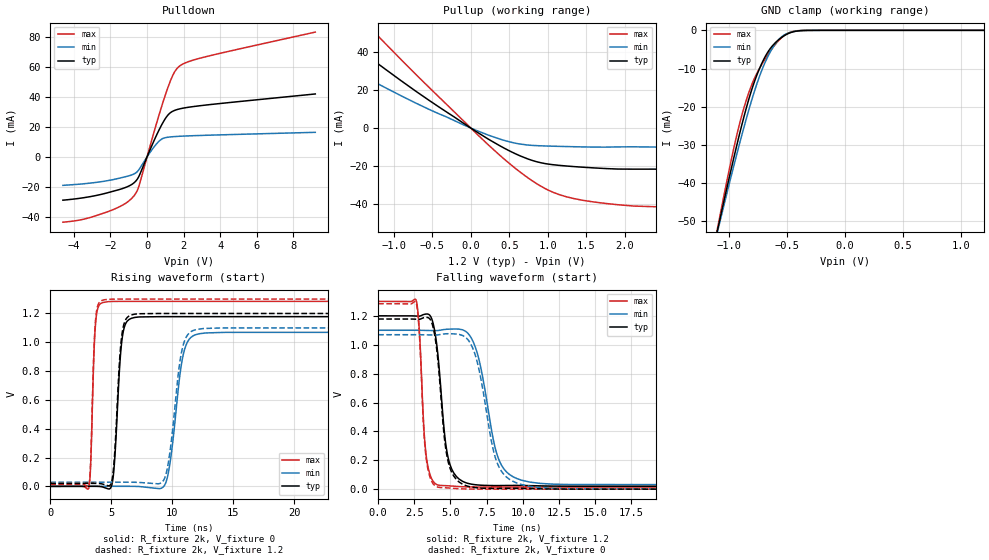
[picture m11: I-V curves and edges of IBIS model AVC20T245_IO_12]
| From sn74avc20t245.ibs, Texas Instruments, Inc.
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[Model]   AVC20T245_IO_12
Model_type  I/O
Vinl=0.385
Vinh=0.845
Enable   Active-Low
Vref =   0
Rref =   2000
Cref =   15p
Vmeas =   0.6
| variable   typ   min   max
C_comp   5.29pF   4.66pF   5.83pF
| C_pullup   5.78pF   3.89pF   7.84pF
| C_pulldown   5.32pF   4.76pF   7.02pF
| C_tri-state   5.29pF   4.66pF   5.83pF
[Temperature Range]   40   100   -40
| Ambient temperature   25   85   -40
[Voltage range]   1.2   1.1   1.3
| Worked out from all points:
|   slope of the pulldown table from 0 to 0.18 V, typ, clamps not added: 34.6 ohm
|   slope of the pullup table from 0 to 0.18 V, typ, clamps not added: 38.6 ohm
|   GND clamp passes 1 mA (typ) near -0.50 V on its own axis
|   rising waveform, R_fixture 2k, V_fixture 0: 20-80 % time 468ps typ, 865ps min, 281ps max; typ from 0 V to 1.18 V
|   falling waveform, R_fixture 2k, V_fixture 1.2: 20-80 % time 670ps typ, 1.21ns min, 399ps max; typ from 1.2 V to 0.02 V
|   rising waveform, R_fixture 2k, V_fixture 1.2: 20-80 % time 463ps typ, 848ps min, 279ps max; typ from 0.02 V to 1.2 V
|   falling waveform, R_fixture 2k, V_fixture 0: 20-80 % time 668ps typ, 1.21ns min, 397ps max; typ from 1.18 V to 0 V
[GND Clamp]
| AVC20T245_IO_12
|   Voltage   I(typ)   I(min)   I(max)
-4.6V     -597.8mA   -546.6mA   -662.5mA
-1.095V   -51.41mA   -51.9mA    -50.81mA
-1.07V    -47.97mA   -48.78mA   -46.93mA
-940mV    -30.76mA   -33.04mA   -28.1mA
-840mV    -18.99mA   -21.8mA    -17.13mA
-775mV    -12.84mA   -15.28mA   -12.1mA
-695mV    -7.204mA   -8.735mA   -7.744mA
-615mV    -3.665mA   -4.111mA   -4.191mA
-545mV    -1.809mA   -1.649mA   -1.862mA
-465mV    -549.4uA   -452.3uA   -430.6uA
-360mV    -50.53uA   -51.18uA   -21.62uA
1.2V      708.7pA    34.3nA     62.33pA
[Pulldown]
| AVC20T245_IO_12
|   Voltage   I(typ)   I(min)   I(max)
-4.6V     -28.79mA   -18.92mA   -43.46mA
-3.415V   -27.06mA   -17.81mA   -41.32mA
-2.03V    -23.44mA   -15.52mA   -35.94mA
-1.165V   -20.28mA   -13.12mA   -30.82mA
-680mV    -16.87mA   -11.13mA   -25.38mA
-435mV    -12.68mA   -8.327mA   -19.06mA
440mV     12.38mA    7.543mA    19.04mA
955mV     24.67mA    12.69mA    39.57mA
1.42V     30.53mA    13.49mA    54.64mA
1.79V     32.04mA    13.78mA    60.61mA
3.17V     34.51mA    14.41mA    66.63mA
9.2V      41.96mA    16.4mA     83.17mA
[Pullup]
| AVC20T245_IO_12
|   Voltage   I(typ)   I(min)   I(max)
-4.6V     40.24mA    7.956mA    186.3mA
-4.08V    45.4mA     8.808mA    167.8mA
-3.73V    53.62mA    9.647mA    154.2mA
-2.685V   79.31mA    16.98mA    111.4mA
-2.57V    75.87mA    21.96mA    106.5mA
-2.565V   75.72mA    49.42mA    106.3mA
-1.845V   53.66mA    37.03mA    75.82mA
-1.36V    38.76mA    26.71mA    55.3mA
575mV     -13.51mA   -7.977mA   -21.19mA
1.01V     -19.08mA   -9.527mA   -32.92mA
1.455V    -20.71mA   -9.971mA   -38.21mA
9.2V      -28.28mA   -12.48mA   -52.65mA
[Ramp]
| AVC20T245_IO_12
| variable   typ   min   max
dV/dt_r   0.72/4.81E-10   0.65/8.80E-10   0.78/2.90E-10
dV/dt_f   0.72/6.78E-10   0.65/1.22E-09   0.78/4.10E-10
R_load = 2k
[Rising Waveform]
| AVC20T245_IO_12
R_fixture =   2k
C_fixture =   0
L_fixture =   0
V_fixture =   0
V_fixture_min = 0
V_fixture_max = 0
|   Time   V(typ)   V(min)   V(max)
0s        18.11nV    102nV      416.8pV
3.155ns   608.7uV    -112.2uV   -13.83mV
3.7ns     442.6uV    152uV      1.117V
4.28ns    -4.064mV   161.8uV    1.276V
5.105ns   34.06mV    467.8uV    1.283V
5.86ns    1.005V     358.8uV    1.284V
6.64ns    1.166V     217.5uV    1.284V
9.455ns   1.178V     21.9mV     1.284V
11.88ns   1.178V     1.052V     1.284V
40ns      1.178V     1.069V     1.284V
[Falling Waveform]
| AVC20T245_IO_12
R_fixture =   2k
C_fixture =   0
L_fixture =   0
V_fixture =   1.2
V_fixture_min = 1.1
V_fixture_max = 1.3
|   Time   V(typ)   V(min)   V(max)
0s        1.2V       1.1V       1.3V
2.635ns   1.198V     1.1V       1.304V
3.305ns   1.212V     1.099V     245.1mV
4.115ns   945.3mV    1.098V     29.65mV
4.675ns   312.6mV    1.106V     24.25mV
5.235ns   111.2mV    1.109V     20.5mV
6.58ns    32.59mV    1.019V     15.04mV
8.275ns   25.01mV    223.6mV    14.53mV
9.915ns   25.68mV    62.19mV    14.51mV
40ns      20.14mV    28.75mV    14.5mV
[Rising Waveform]
| AVC20T245_IO_12
R_fixture =   2k
C_fixture =   0
L_fixture =   0
V_fixture =   1.2
V_fixture_min = 1.1
V_fixture_max = 1.3
|   Time   V(typ)   V(min)   V(max)
0s        20.14mV    28.74mV    14.5mV
3.155ns   20.71mV    28.68mV    2.227mV
3.69ns    20.46mV    28.94mV    1.131V
4.235ns   16.88mV    28.9mV     1.291V
5.075ns   49.5mV     29.12mV    1.299V
5.825ns   1.021V     28.88mV    1.3V
6.61ns    1.189V     28.64mV    1.3V
9.375ns   1.2V       55.91mV    1.3V
11.74ns   1.2V       1.083V     1.3V
40ns      1.2V       1.1V       1.3V
[Falling Waveform]
| AVC20T245_IO_12
R_fixture =   2k
C_fixture =   0
L_fixture =   0
V_fixture =   0
V_fixture_min = 0
V_fixture_max = 0
|   Time   V(typ)   V(min)   V(max)
0s        1.178V     1.069V     1.284V
2.635ns   1.177V     1.069V     1.287V
3.3ns     1.189V     1.068V     230.3mV
4.095ns   927.4mV    1.068V     15.25mV
4.65ns    297mV      1.076V     9.628mV
5.22ns    92.15mV    1.075V     5.452mV
6.67ns    11.31mV    942.6mV    370.1uV
8.3ns     5.043mV    165.5mV    26.33uV
9.85ns    5.41mV     33.86mV    7.037uV
40ns      16.35nV    4.569uV    -1.054nV
